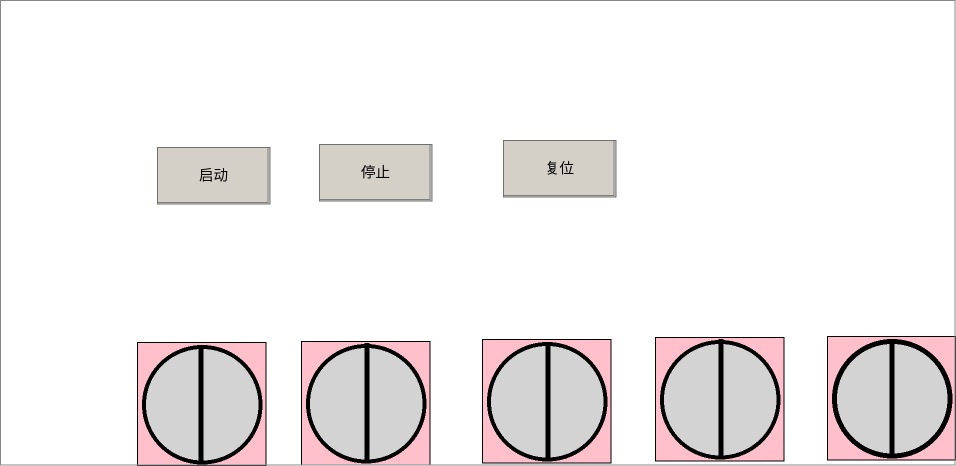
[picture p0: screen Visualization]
VISUALIZATION Visualization  // 956x466
    Textfield (137,342 129x124), invisible if: MAIN.fbVisus.ArrAxisNotMoving[1]
    Ellipse (142,345 120x119)
    Textfield (301,341 129x124), invisible if: MAIN.fbVisus.ArrAxisNotMoving[2]
    Ellipse (306,344 120x119)
    Textfield (482,339 129x124), invisible if: MAIN.fbVisus.ArrAxisNotMoving[3]
    Ellipse (487,342 120x119)
    Textfield (655,337 129x124), invisible if: MAIN.fbVisus.ArrAxisNotMoving[4]
    Ellipse (660,340 120x119)
    Textfield (827,336 129x124), invisible if: MAIN.fbVisus.ArrAxisNotMoving[5]
    Ellipse (832,339 120x119)
    Polyline (201,464) (201,346)
        p2858320360: MAIN.fbVisus.ArrAxisPosition[1]
    Polyline (367,461) (367,343)
        p2858320360: MAIN.fbVisus.ArrAxisPosition[2]
    Polyline (548,461) (548,343)
        p2858320360: MAIN.fbVisus.ArrAxisPosition[3]
    Polyline (721,457) (721,339)
        p2858320360: MAIN.fbVisus.ArrAxisPosition[4]
    Polyline (892,458) (892,340)
        p2858320360: MAIN.fbVisus.ArrAxisPosition[5]
    Button (157,147 113x57), "启动"
        toggle MAIN.bStart
    Button (319,144 113x57), "停止"
        toggle MAIN.bStop
    Button (503,140 113x57), "复位"
        toggle MAIN.bReset
END_VISUALIZATION
